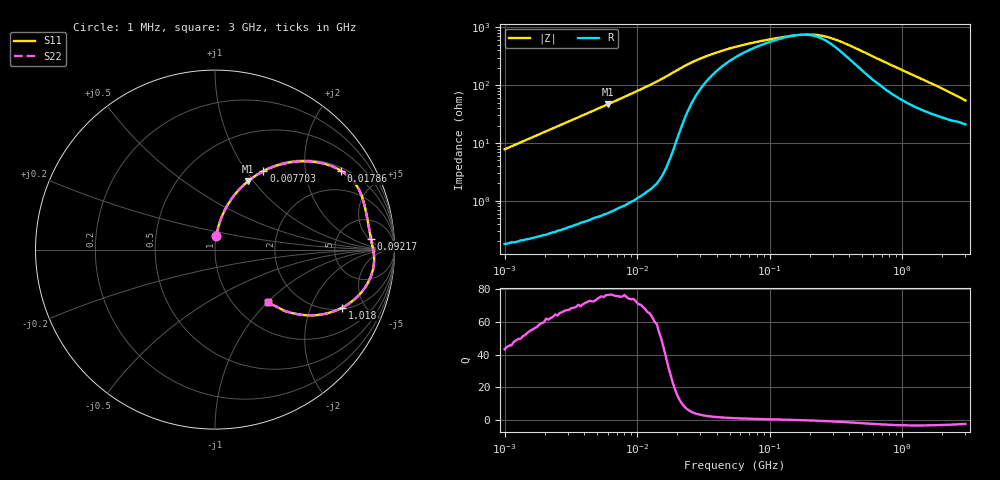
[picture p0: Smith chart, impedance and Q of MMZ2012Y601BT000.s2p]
! S-parameter Generated by TDK Corporation
! Copyright(C) 2016 TDK Corporation.
! All Rights Reserved.
! TDK P/N: MMZ2012Y601BT000 (Chip Beads)
! Property: |Z|=600¶ at 100MHz
! Size(LxWxT): 2x1.25x0.85mm, 0.079x0.049x0.033inches
! Model Type: s2p (Touchstone File Format Version 1.0)
! Frequency: DC=Yes Start=1MHz Stop=3000MHz 202points Log-sweep
! Note: This model was converted from impedance.
! Model Generated on May. 16, 2016
! Hash(MD5):
! Port Assignments:
!  1 ---@@@--- 2
! Applicable Conditions:
!  Temperature = 25 degC
!  DC Bias Current = 0 A
!  Small Signal Operation
! Terms and conditions regarding TDK Simulation Models
! (1)This simulation model is being provided solely for informational purposes. Please refer to the specifications of the products in terms of detailed characteristics of such products.
! (2)In no event shall TDK Corporation of any of its subsidiaries be liable for any loss or damage arising, directly or indirectly,
!  From any information contained in this simulation model, including, but not limited to loss or damages arising from any inaccuracies, omissions or errors in connection with such information.
! (3)Any and all copyrights on this simulation model are owned by TDK Corporation.
!  Duplication or redistribution of this simulation model without prior written permission from TDK Corporation is prohibited.
! (4)This simulation model is subject to any modification or change without any prior notice.
! (5)Neither TDK Corporation nor any of its subsidiaries shall make any warranty, express or implied,
!  Including but not limited to the correctness, implied warranties of merchantability and fitness for a particular purpose with respect to this simulation models.
! (6)The use of this simulation model shall be deemed to have consented to the terms and conditions hereof.
# MHz S MA R 50
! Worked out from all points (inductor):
!   201 points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, 1 MHz to 3 GHz, reference 50 ohm
!   read as one part in series: L = 1.24 uH near 1.041 MHz
!   highest Q = 76.4 at 6.058 MHz (marker M1), where L = 1.24 uH
!   self-resonance near 167.6 MHz
!   S11 on the Smith chart (normalised r, x): 1 MHz: 1.00, +0.16; 7.703 MHz: 1.02, +1.21; 17.86 MHz: 1.11, +3.12; 92.17 MHz: 12, +6; 1.018 GHz: 2.08, -3.42; 3 GHz: 1.42, -1.00
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1  0.07747 84.2  0.9952 -4.4  0.9952 -4.4  0.07747 84.2
2.055611  0.1572 80.0  0.985 -9.0  0.985 -9.0  0.1572 80.0
3.900413  0.2883 72.4  0.9535 -16.8  0.9535 -16.8  0.2883 72.4
6.058321  0.4243 64.1  0.9 -25.1  0.9 -25.1  0.4243 64.1
7.703107  0.5134 58.4  0.8514 -30.9  0.8514 -30.9  0.5134 58.4
11.04425  0.6569 48.1  0.7445 -41.1  0.7445 -41.1  0.6569 48.1
14.61624  0.7647 39.1  0.6304 -49.9  0.6304 -49.9  0.7647 39.1
17.85516  0.8285 32.0  0.5308 -55.9  0.5308 -55.9  0.8285 32.0
20.95589  0.8599 26.3  0.445 -59.0  0.445 -59.0  0.8599 26.3
25.59965  0.8702 20.3  0.3532 -58.6  0.3532 -58.6  0.8702 20.3
35.26298  0.8668 13.7  0.2594 -52.5  0.2594 -52.5  0.8668 13.7
54.77226  0.8659 8.2  0.1887 -40.8  0.1887 -40.8  0.8659 8.2
92.16659  0.8703 4.0  0.1452 -24.8  0.1452 -24.8  0.8703 4.0
149.005  0.879 0.8  0.1218 -5.9  0.1218 -5.9  0.879 0.8
213.6344  0.886 -1.9  0.1182 14.3  0.1182 14.3  0.886 -1.9
260.9752  0.8885 -3.7  0.1269 26.7  0.1269 26.7  0.8885 -3.7
318.8066  0.8889 -5.8  0.146 37.6  0.146 37.6  0.8889 -5.8
515.4121  0.8726 -12.1  0.234 51.2  0.234 51.2  0.8726 -12.1
800.5644  0.8245 -19.7  0.3567 51.2  0.3567 51.2  0.8245 -19.7
1017.911  0.7795 -24.5  0.4346 48.0  0.4346 48.0  0.7795 -24.5
1782.824  0.6176 -36.2  0.6205 36.0  0.6205 36.0  0.6176 -36.2
3000  0.4156 -44.7  0.7629 22.5  0.7629 22.5  0.4156 -44.7
